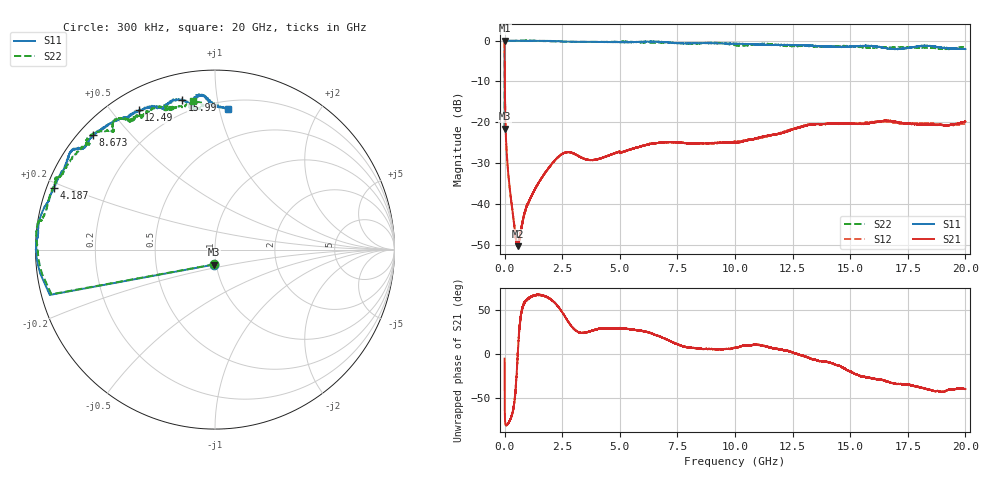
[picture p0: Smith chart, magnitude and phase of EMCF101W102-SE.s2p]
!EMCF101W102
!Johanson Technology Inc.
!www.johansontechnology.com
!Test Board Conditions:
!Substrate Type  RO4350B
!Substrate Thickness  6.6 mil
!Substrate Dk  3.66
!TL Type: GCPW
!TL Trace Width  13 mil
!TL Gap  7.5 mil
!PART MODE SINGLE ENDED (AKA BYPASS)
!DUT TOPOLOGY	SERIES-SHUNT
# MHz S  dB  R 50
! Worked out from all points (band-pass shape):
!   20001 points, 300 kHz to 20 GHz, reference 50 ohm
!   highest |S21| = -0.02 dB at 300 kHz (marker M1); lowest = -50.3 dB at 573.3 MHz (marker M2)
!   |S21| within 3 dB of the highest: start of sweep to 3.515 MHz
!   lowest |S11| = -21.6 dB at 300 kHz (marker M3), VSWR 1.18, Z = 48.8 - j8.2 ohm
!   |S11| at or under -10 dB: start of sweep to 1.246 MHz
!   |S22| runs from -21.7 to 0.0 dB; largest |S21 - S12| = 0.0049
!   S11 on the Smith chart (normalised r, x): 300 kHz: 0.98, -0.16; 4.187 GHz: 0.02, +0.18; 8.673 GHz: 0.04, +0.39; 12.49 GHz: 0.08, +0.59; 15.99 GHz: 0.13, +0.79; 20 GHz: 0.25, +1.06
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0.3  -21.56 -93.3  -0.02 -5.3  -0.01 -5.3  -21.69 -93.4
101.298  -0.05 -178.5  -28.45 -80.4  -28.42 -80.4  -0.12 -178.4
165.298  -0.02 -179.9  -32.92 -78.3  -32.86 -78.2  -0.12 -179.6
441.293  -0.04 178.2  -46.22 -49.7  -46.22 -51.8  -0.04 177.3
573.291  -0.04 177.4  -50.29 -0.1  -49.96 1.7  -0.02 176.2
1009.285  -0.06 176.5  -39.97 62.9  -40.10 62.6  -0.01 172.0
1909.271  -0.07 170.3  -31.21 63.6  -31.11 63.8  -0.16 170.5
2618.261  -0.24 165.1  -27.41 42.8  -27.40 42.3  -0.25 168.2
3334.25  -0.29 163.1  -28.62 24.0  -28.61 24.1  -0.27 163.4
4187.237  -0.34 159.2  -28.75 29.0  -28.75 29.0  -0.29 158.4
6667.2  -0.29 144.9  -25.04 20.8  -24.99 20.4  -0.46 149.7
7864.182  -0.69 141.7  -25.09 8.0  -25.05 8.4  -0.69 140.3
8673.17  -0.60 137.0  -25.14 5.8  -25.17 5.4  -0.59 140.2
10000.15  -0.79 130.7  -24.90 7.1  -24.71 7.4  -1.14 131.3
12486.11  -1.06 118.7  -21.77 1.8  -21.61 2.1  -1.39 122.4
13334.1  -1.27 113.1  -20.56 -5.8  -20.45 -6.3  -1.40 119.1
14433.08  -1.53 110.0  -20.34 -12.7  -20.42 -12.6  -1.39 117.4
15989.06  -1.39 102.5  -20.02 -27.7  -19.92 -29.3  -1.74 106.6
16667.05  -1.98 99.1  -19.60 -31.6  -19.93 -32.5  -1.68 109.1
17245.04  -1.99 98.8  -20.15 -34.1  -20.22 -33.1  -1.71 108.0
18609.02  -1.42 93.7  -20.55 -41.7  -20.35 -42.7  -1.81 95.2
20000  -2.04 84.7  -19.80 -39.7  -20.12 -38.8  -1.54 98.3
